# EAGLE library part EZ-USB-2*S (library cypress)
Microcontroller with USB port
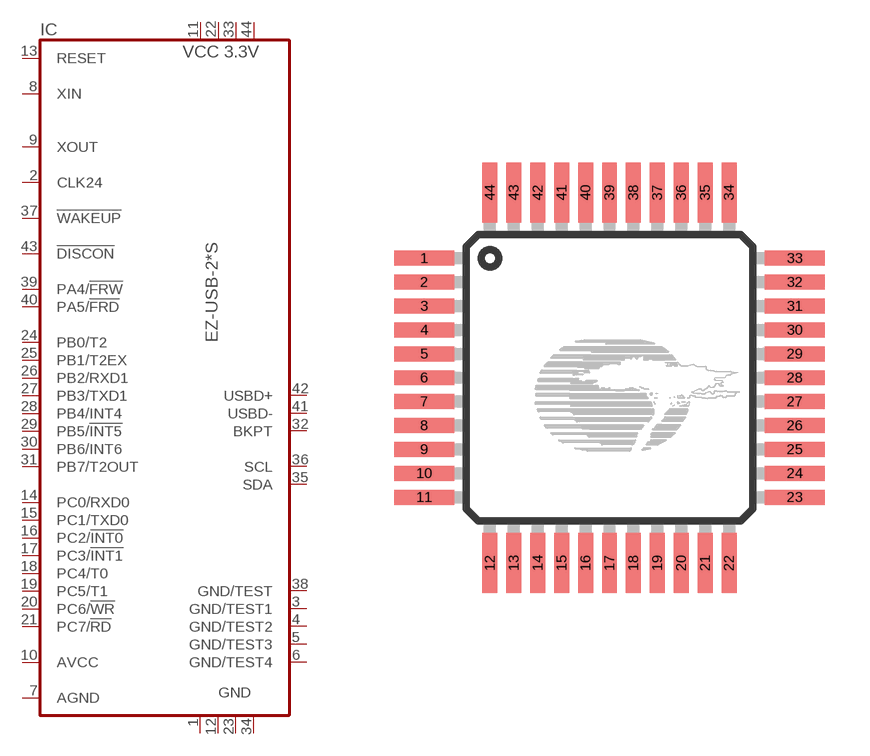
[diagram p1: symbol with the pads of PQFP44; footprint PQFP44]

Designator prefix IC

## EZ-USB-2121S (OC_FARNELL: unknown; OC_NEWARK: unknown), EZ-USB-2122S (OC_FARNELL: unknown; OC_NEWARK: unknown), EZ-USB-2131S (OC_FARNELL: unknown; OC_NEWARK: unknown)  [PQFP44]
1  GND  pwr
2  CLK24  out
3  GND/TEST1  pwr
4  GND/TEST2  pwr
5  GND/TEST3  pwr
6  GND/TEST4  pwr
7  AGND  pwr
8  XIN  in
9  XOUT  out
10  AVCC  pwr
11  VCC3.3  pwr
12  GND  pwr
13  RESET  in
14  PC0/RXD0
15  PC1/TXD0
16  PC2/!INT0
17  PC3/!INT1
18  PC4/T0
19  PC5/T1
20  PC6/!WR
21  PC7/!RD
22  VCC3.3  pwr
23  GND  pwr
24  PB0/T2
25  PB1/T2EX
26  PB2/RXD1
27  PB3/TXD1
28  PB4/INT4
29  PB5/!INT5
30  PB6/INT6
31  PB7/T2OUT
32  BKPT  out
33  VCC3.3  pwr
34  GND  pwr
35  SDA  oc
36  SCL  oc
37  !WAKEUP  in
38  GND/TEST  pwr
39  PA4/!FRW
40  PA5/!FRD
41  USBD-  hiz
42  USBD+  hiz
43  !DISCON  out
44  VCC3.3  pwr

## Footprint PQFP44 (pad centres in mm)
Plastic Quad Flat Package
smd 2 x 0.5: 1 -6.2,4; 2 -6.2,3.2; 3 -6.2,2.4; 4 -6.2,1.6; 5 -6.2,0.8; 6 -6.2,0; 7 -6.2,-0.8; 8 -6.2,-1.6; 9 -6.2,-2.4; 10 -6.2,-3.2; 11 -6.2,-4; 23 6.2,-4; 24 6.2,-3.2; 25 6.2,-2.4; 26 6.2,-1.6; 27 6.2,-0.8; 28 6.2,0; 29 6.2,0.8; 30 6.2,1.6; 31 6.2,2.4; 32 6.2,3.2; 33 6.2,4
smd 0.5 x 2: 12 -4,-6.2; 13 -3.2,-6.2; 14 -2.4,-6.2; 15 -1.6,-6.2; 16 -0.8,-6.2; 17 0,-6.2; 18 0.8,-6.2; 19 1.6,-6.2; 20 2.4,-6.2; 21 3.2,-6.2; 22 4,-6.2; 34 4,6.2; 35 3.2,6.2; 36 2.4,6.2; 37 1.6,6.2; 38 0.8,6.2; 39 0,6.2; 40 -0.8,6.2; 41 -1.6,6.2; 42 -2.4,6.2; 43 -3.2,6.2; 44 -4,6.2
